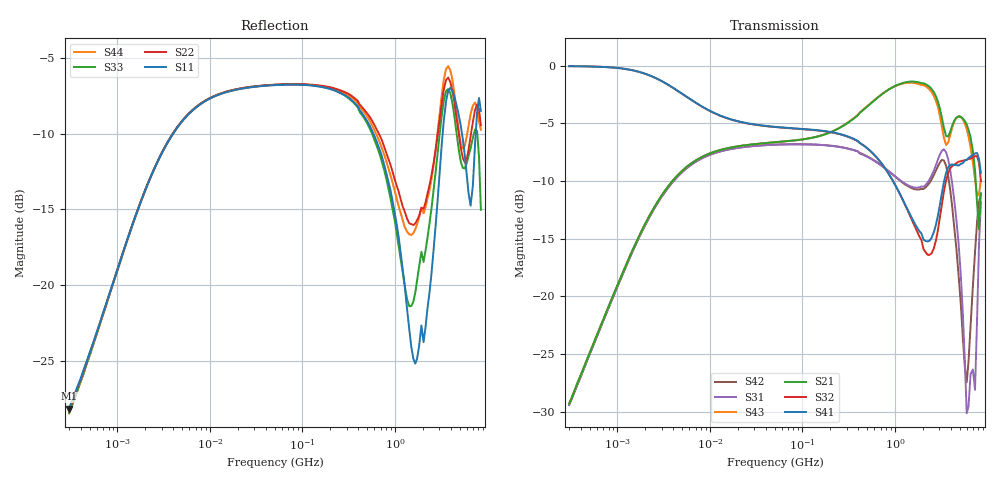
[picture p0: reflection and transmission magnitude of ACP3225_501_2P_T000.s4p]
! S-parameter Generated by TDK Corporation
! Copyright(C) 2018 TDK Corporation.
! All Rights Reserved.
! TDK P/N: ACP3225-501-2P-T000 (Common Mode Filter)
! Property: |Zc|=500¶ at 100MHz
! Size(LxWxT): 3.2x2.5x1.9mm, 0.126x0.098x0.075inches
! Model Type: s4p (Touchstone File Format Version 1.0)
! Frequency: DC=Yes Start=0.3MHz Stop=8500MHz 202points Log-sweep
! Model Generated on Aug. 28, 2018
! Port Assignments:
!  1 ---@@@--- 4
!  2 ---@@@--- 3
! Applicable Conditions:
!  Temperature = 25 degC
!  DC Bias Current = 0 A
!  Small Signal Operation
! Terms and conditions regarding TDK Simulation Models
! (1)This simulation model is being provided solely for informational purposes. Please refer to the specifications of the products in terms of detailed characteristics of such products.
! (2)In no event shall TDK Corporation of any of its subsidiaries be liable for any loss or damage arising, directly or indirectly,
!  From any information contained in this simulation model, including, but not limited to loss or damages arising from any inaccuracies, omissions or errors in connection with such information.
! (3)Any and all copyrights on this simulation model are owned by TDK Corporation.
!  Duplication or redistribution of this simulation model without prior written permission from TDK Corporation is prohibited.
! (4)This simulation model is subject to any modification or change without any prior notice.
! (5)Neither TDK Corporation nor any of its subsidiaries shall make any warranty, express or implied,
!  Including but not limited to the correctness, implied warranties of merchantability and fitness for a particular purpose with respect to this simulation models.
! (6)The use of this simulation model shall be deemed to have consented to the terms and conditions hereof.
# Hz S MA R 50
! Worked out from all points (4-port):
!   201 points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, 300 kHz to 8.5 GHz, reference 50 ohm
!   strongest paths, dB at 300 kHz, 3.892 MHz, 50.5 MHz, 655.2 MHz, 8.5 GHz:
!     S41: 0.0, -1.8, -5.3, -8.1, -9.3
!     S32: 0.0, -1.9, -5.3, -8.1, -10.0
!     S21: -29.3, -10.0, -6.6, -2.7, -11.1
!     S43: -29.3, -10.0, -6.6, -2.7, -9.9
!     S31: -29.4, -10.1, -6.8, -8.5, -11.9
!     S42: -29.4, -10.1, -6.8, -8.4, -11.2
!   lowest |S11| = -28.2 dB at 300 kHz (marker M1), VSWR 1.08, Z = 49.9 + j3.91 ohm
!   |S11| at or under -10 dB: start of sweep to 3.987 MHz; 586.7 MHz to 3.284 GHz (2.697 GHz wide, 139 % of centre); 5.312 GHz to 7.476 GHz (2.164 GHz wide, 33.8 % of centre)
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300000  0.03905 88.5  0.03431 85.6  0.03369 -94.3  0.9973 -1.9
        0.03419 85.5  0.03873 87.0  0.9965 -1.9  0.03363 -94.6
        0.03373 -94.5  0.9964 -1.9  0.03772 86.5  0.03421 85.8
        0.9964 -1.9  0.03392 -94.1  0.03418 85.6  0.03767 86.7
1.091e7  0.419 19.9  0.4224 21.5  0.4167 -160.6  0.627 -14.8
         0.4223 21.5  0.4205 20.1  0.6258 -14.9  0.4167 -160.3
         0.4166 -160.6  0.6257 -14.9  0.4202 19.9  0.4225 21.5
         0.6268 -14.8  0.4166 -160.3  0.4224 21.5  0.4189 20.1
1.157143e9  0.1267 -66.5  0.8372 -7.5  0.3178 73.7  0.2749 -86.8
            0.8373 -7.4  0.1915 -38.5  0.2725 -89.8  0.316 90.9
            0.3179 73.7  0.2727 -89.8  0.1208 -54.6  0.8332 -10.5
            0.2738 -87.2  0.3158 90.6  0.8332 -10.5  0.1725 -35.5
2.03972e9  0.06475 7.6  0.8393 -32.5  0.2986 39.1  0.1735 -122.8
           0.84 -32.5  0.1787 -25.2  0.1597 -138.1  0.2907 55.6
           0.2985 39.1  0.1602 -138.2  0.1193 -6.8  0.8254 -37.4
           0.1763 -122.8  0.2924 55.7  0.8248 -37.5  0.1727 -5.7
3.575798e9  0.4058 -59.5  0.4953 -57.9  0.4202 -39.6  0.3426 120.5
            0.4956 -58.0  0.4769 -78.2  0.3172 90.6  0.3715 -35.7
            0.4223 -39.4  0.3181 90.9  0.4382 -86.2  0.4538 -61.6
            0.3436 119.9  0.3686 -35.8  0.4535 -61.6  0.5186 -63.4
5.973799e9  0.2325 -90.8  0.5565 -85.0  0.03093 -92.9  0.3937 -10.4
            0.5558 -85.1  0.2602 -73.0  0.3884 -23.9  0.05032 139.9
            0.03109 -91.5  0.3912 -23.8  0.2532 -74.3  0.5319 -98.5
            0.3913 -10.7  0.04239 142.6  0.5319 -98.5  0.3098 -70.3
8.5e9  0.3765 -101.2  0.2814 -69.3  0.2559 -19.5  0.3495 -129.2
       0.2801 -69.6  0.337 -122.3  0.3154 -115.6  0.2774 -28.0
       0.2555 -19.1  0.3162 -116.0  0.1773 -97.3  0.319 -112.5
       0.3432 -129.6  0.2765 -27.4  0.3199 -113.0  0.3264 -73.4
